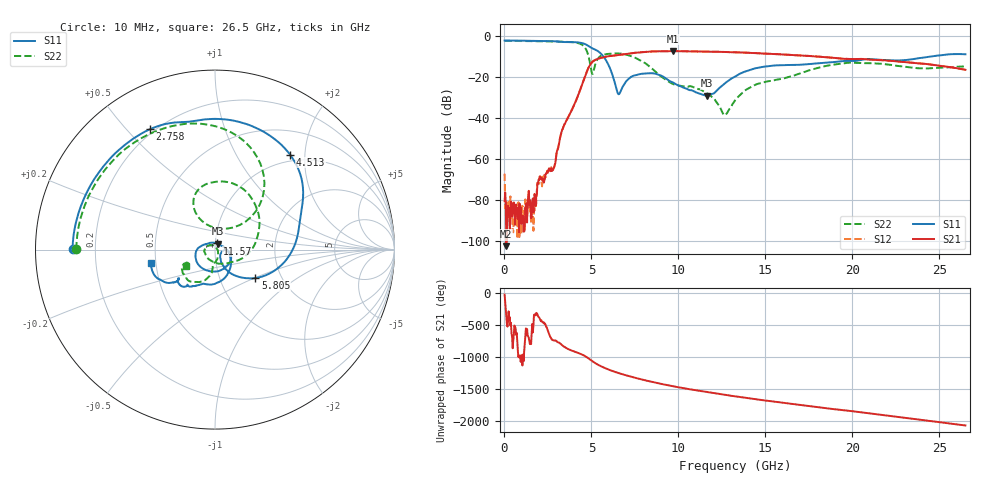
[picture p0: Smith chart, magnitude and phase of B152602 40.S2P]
!  2-Port S-parameters saved by WinCal
! VAR MeasName=S-Parameters (CALIBRATED_DATA) read from VNA (N5242A)
! VAR MeasDate=2016-1-5 16:31:55
! VAR NAME=B152602 40
! VAR FILENAME=B152602 40.S2P
! VAR DATE=2016-1-5 16:31:55
! VAR PHYS_PORTS=1,2
# Hz S DB R 50
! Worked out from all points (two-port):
!   801 points, 10 MHz to 26.5 GHz, reference 50 ohm
!   highest |S21| = -7.21 dB at 9.679 GHz (marker M1); lowest = -102.6 dB at 109.3 MHz (marker M2)
!   |S21| within 3 dB of the highest: 5.701 GHz to 18.48 GHz (12.78 GHz wide, 106 % of centre)
!   lowest |S11| = -29.0 dB at 11.67 GHz (marker M3), VSWR 1.07, Z = 51.4 + j3.33 ohm
!   |S11| at or under -10 dB: 5.707 GHz to 24.39 GHz (18.68 GHz wide, 124 % of centre)
!   |S22| runs from -38.6 to -2.2 dB; largest |S21 - S12| = 0.0029
!   S11 on the Smith chart (normalised r, x): 10 MHz: 0.12, +0.00; 2.758 GHz: 0.18, +0.58; 4.513 GHz: 0.88, +1.71; 5.805 GHz: 1.48, -0.51; 11.57 GHz: 1.02, +0.07; 26.5 GHz: 0.47, -0.08
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1e7  -2.01 179.7  -80.60 -17.3  -67.15 109.1  -2.24 179.8
1.093375e8  -2.01 177.7  -102.56 28.7  -81.05 31.9  -2.24 178.3
1.698738e9  -2.20 144.7  -80.95 25.4  -85.42 78.3  -2.36 153.3
2.029862e9  -2.23 137.2  -68.49 -34.7  -68.46 -37.3  -2.39 147.7
2.758338e9  -2.35 118.6  -65.56 -2.9  -65.46 -1.1  -2.47 134.0
3.354362e9  -2.77 101.5  -45.18 -99.3  -45.22 -99.3  -2.60 120.3
4.447075e9  -3.28 55.6  -24.00 126.8  -24.01 126.8  -4.03 75.5
4.5133e9  -3.42 51.6  -22.43 118.2  -22.44 118.3  -4.43 70.6
5.076212e9  -5.96 19.6  -12.32 16.7  -12.33 16.8  -18.33 89.5
5.804688e9  -11.22 -35.2  -10.03 -89.4  -10.01 -89.3  -8.76 99.4
6.566275e9  -28.31 -28.5  -9.10 -164.9  -9.10 -164.9  -8.36 75.1
7.758325e9  -18.51 -70.7  -7.81 104.3  -7.80 104.3  -11.53 23.1
8.851038e9  -18.71 -159.5  -7.32 35.4  -7.31 35.2  -18.62 -36.4
9.67885e9  -22.51 161.4  -7.21 -9.9  -7.22 -9.9  -23.25 -98.9
1.156626e10  -28.95 73.5  -7.43 -99.1  -7.44 -99.0  -27.49 147.5
1.16656e10  -28.98 65.4  -7.47 -103.3  -7.46 -103.2  -27.89 142.0
1.265898e10  -23.09 -6.2  -7.63 -144.6  -7.65 -144.5  -38.56 37.0
1.3255e10  -19.68 -32.8  -7.79 -168.1  -7.79 -168.1  -31.32 -50.7
1.547354e10  -14.31 -92.6  -8.66 109.2  -8.61 109.2  -21.55 -97.6
1.769208e10  -13.43 -113.3  -9.70 32.4  -9.67 32.5  -16.21 -102.5
2.209604e10  -11.66 -141.6  -11.90 -111.3  -11.85 -111.6  -13.83 -153.0
2.65e10  -8.76 -168.0  -16.34 96.6  -16.35 96.3  -14.69 -150.0
